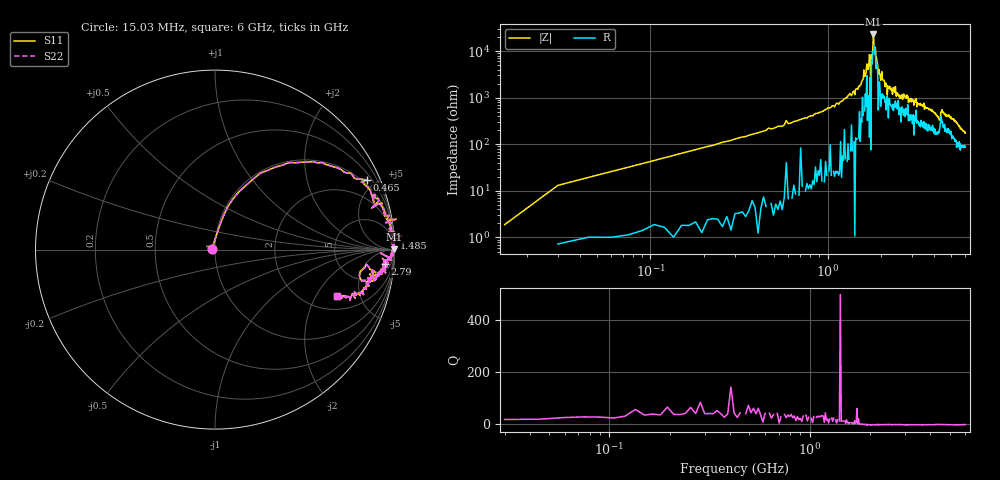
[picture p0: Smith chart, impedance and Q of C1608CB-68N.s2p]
!	Network	Analyzer	HP8753E.07.74:	Oct	30	2002	Serial	No.	JP38451487
!	Hewlett-Packard
!	7	Sep	2009	9:48:31
!	Frequency	S11	S21	S12	S22
#	HZ	S	RI	R	50
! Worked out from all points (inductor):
!   400 points, 15.03 MHz to 6 GHz, reference 50 ohm
!   read as one part in series: L = 68.5 nH near 45.03 MHz
!   highest |Z| = 22.7 kohm at 1.815 GHz (marker M1)
!   self-resonance near 1.77 GHz
!   S11 on the Smith chart (normalised r, x): 15.03 MHz: 0.97, +0.01; 465 MHz: 0.74, +4.46; 1.485 GHz: -0, +30; 2.79 GHz: 10, -17; 6 GHz: 2.77, -3.02
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1.502992e7  -0.0169 0.00529  1.02 -0.00529  1.02 -0.00529  -0.0169 0.00529
3.002985e7  0.0235 0.127  0.976 -0.127  0.976 -0.127  0.0235 0.127
9.002955e7  0.138 0.327  0.862 -0.327  0.862 -0.327  0.138 0.327
4.650277e8  0.848 0.389  0.152 -0.389  0.152 -0.389  0.848 0.389
1.020025e9  0.966 0.16  0.0339 -0.16  0.0339 -0.16  0.966 0.16
1.485023e9  0.998 0.0661  0.00183 -0.0661  0.00183 -0.0661  0.998 0.0661
1.695022e9  0.993 0.0236  0.00736 -0.0236  0.00736 -0.0236  0.993 0.0236
1.725021e9  1 0.0118  0.000336 -0.0118  0.000336 -0.0118  1 0.0118
1.740021e9  0.994 0.0135  0.00629 -0.0135  0.00629 -0.0135  0.994 0.0135
1.755021e9  0.993 0.0632  0.00711 -0.0632  0.00711 -0.0632  0.993 0.0632
1.770021e9  0.991 0.00726  0.00937 -0.00726  0.00937 -0.00726  0.991 0.00726
1.785021e9  0.989 -0.00909  0.0112 0.00909  0.0112 0.00909  0.989 -0.00909
1.815021e9  1 0.00226  -0.00378 -0.00226  -0.00378 -0.00226  1 0.00226
1.93502e9  0.994 -0.0306  0.00626 0.0306  0.00626 0.0306  0.994 -0.0306
2.01002e9  0.986 -0.0308  0.0143 0.0308  0.0143 0.0308  0.986 -0.0308
2.175019e9  0.922 -0.0194  0.0779 0.0194  0.0779 0.0194  0.922 -0.0194
2.415018e9  0.97 -0.0475  0.0298 0.0475  0.0298 0.0475  0.97 -0.0475
2.790016e9  0.947 -0.0813  0.0526 0.0813  0.0526 0.0813  0.947 -0.0813
3.015015e9  0.959 -0.0962  0.0409 0.0962  0.0409 0.0962  0.959 -0.0962
4.00501e9  0.898 -0.166  0.102 0.166  0.102 0.166  0.898 -0.166
5.010005e9  0.853 -0.189  0.147 0.189  0.147 0.189  0.853 -0.189
6e9  0.677 -0.259  0.323 0.259  0.323 0.259  0.677 -0.259
